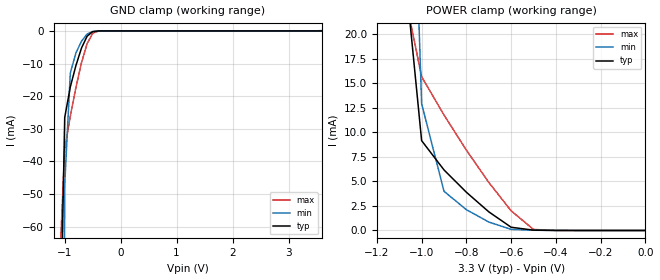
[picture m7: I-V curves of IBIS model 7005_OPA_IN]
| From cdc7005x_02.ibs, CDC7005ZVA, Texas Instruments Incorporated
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| OPA IN
[Model]   7005_OPA_IN
Model_type  Input
Polarity   Non-Inverting
Vinl = 1.6V   | differntial input. Levels set to VCC/2 +/- 50mV
Vinh = 1.7V
| variable   typ   min   max
C_comp   0.52p   NA   NA
[Temperature Range]   27   125   -20
[Voltage range]   3.3   3.0   3.6
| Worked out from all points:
|   GND clamp passes 1 mA (typ) near -0.56 V on its own axis
|   POWER clamp passes 1 mA (typ) near -0.64 V on its own axis
|Process range|   nominal   weak   strong
[POWER Clamp]
|   27C:3.3V:nominal   125C:3.0V:weak  -20C:3.6V:strong
|  Voltage   I(typ)   I(min)   I(max)
-3.6V     4.178A     3.281A     5.394A
-1.1V     32.36mA    81.72mA    26.85mA
-1V       9.154mA    12.92mA    15.67mA
-900mV    6.171mA    3.99mA     11.76mA
-800mV    3.895mA    2.119mA    8.185mA
-700mV    1.902mA    861.1uA    4.902mA
-600mV    327.8uA    109.2uA    1.999mA
-500mV    33.36uA    25.15uA    97.83uA
-400mV    3.107uA    3.538uA    10.35uA
0V        86.16pA    1.105nA    73.5pA
[GND Clamp]
|   27C:3.3V:nominal   125C:3.0V:weak  -20C:3.6V:strong
|  Voltage   I(typ)   I(min)   I(max)
-3.6V     -12.56A    -9.883A    -16.21A
-1.1V     -114.4mA   -281.6mA   -75.44mA
-1V       -26.54mA   -47.04mA   -36.21mA
-900mV    -17.17mA   -12.9mA    -26.15mA
-800mV    -10.61mA   -6.755mA   -17.33mA
-700mV    -5.244mA   -3.141mA   -9.743mA
-600mV    -1.619mA   -969.8uA   -3.911mA
-500mV    -219.4uA   -175uA     -731.5uA
-400mV    -14.85uA   -21.96uA   -44.51uA
3.6V      144.4nA    109.2uA    73.5pA
